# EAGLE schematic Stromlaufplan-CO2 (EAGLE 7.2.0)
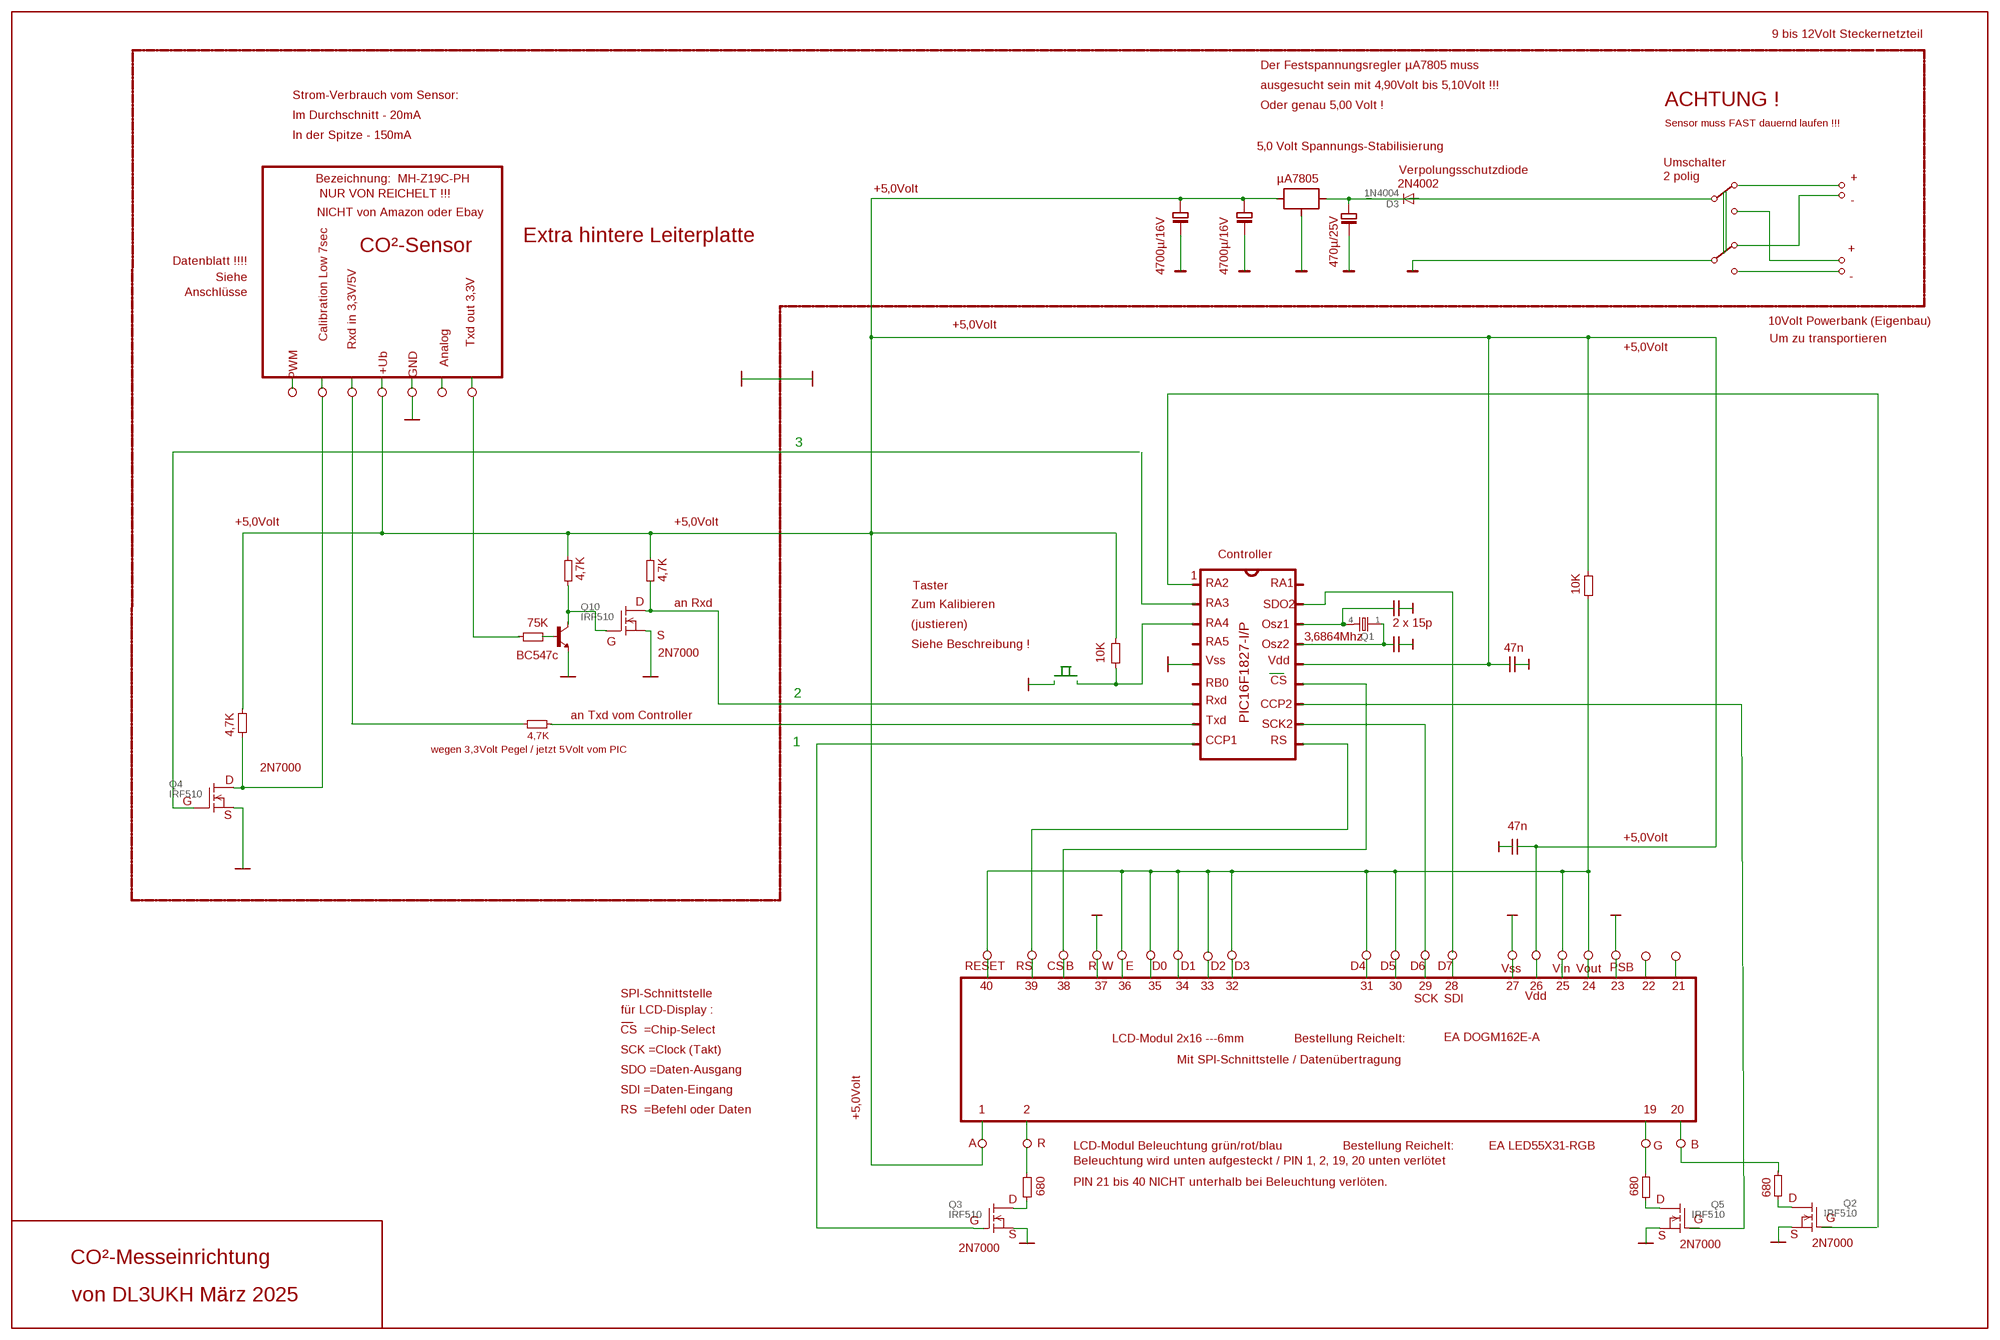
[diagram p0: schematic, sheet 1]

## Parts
D3  1N4004  [DO41-10]
Q1  86SMX  [86SMX]
Q2  IRF510  [TO220]
Q3  IRF510  [TO220]
Q4  IRF510  [TO220]
Q5  IRF510  [TO220]
Q10  IRF510  [TO220]

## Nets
N$7: Q4.1(G)
N$21: Q10.3(S)
N$33: Q10.1(G)
N$39: Q10.2(D)
N$44: Q1.4
N$45: Q1.1
N$47: D3.C
N$56: Q3.2(D)
N$58: Q3.3(S)
N$59: Q3.1(G)
N$60: Q5.1(G)
N$61: Q5.2(D)
N$63: Q5.3(S)
N$64: Q2.2(D)
N$85: Q4.3(S)
N$86: Q4.2(D)
N$87: D3.A
N$96: Q2.3(S)
N$97: Q2.1(G)

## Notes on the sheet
- 9 bis 12Volt Steckernetzteil
- Der Festspannungsregler µA7805 muss
- ausgesucht sein mit 4,90Volt bis 5,10Volt !!!
- Strom-Verbrauch vom Sensor:
- Oder genau 5,00 Volt ! | ACHTUNG !
- Im Durchschnitt - 20mA
- Sensor muss FAST dauernd laufen !!!
- In der Spitze - 150mA
- 5,0 Volt Spannungs-Stabilisierung
- Umschalter
- Bezeichnung:  MH-Z19C-PH | Verpolungsschutzdiode
- µA7805 | 2 polig | +
- NUR VON REICHELT !!! | 2N4002
- +5,0Volt
- -
- NICHT von Amazon oder Ebay
- Calibration Low 7sec
- CO²-Sensor | Extra hintere Leiterplatte
- +
- Datenblatt !!!!
- Rxd in 3,3V/5V | 470µ/25V
- Siehe | 4700µ/16V | 4700µ/16V
- Txd out 3,3V | -
- Anschlüsse
- 10Volt Powerbank (Eigenbau)
- Analog | +5,0Volt
- Um zu transportieren
- PWM | +Ub | GND | +5,0Volt
- 3
- +5,0Volt | +5,0Volt
- Controller
- 4,7K | 4,7K | 1
- Taster | RA2 | RA1
- 10K
- D | an Rxd | Zum Kalibieren | RA3 | SDO2
- 75K | (justieren) | RA4 | Osz1 | 2 x 15p
- S | 3,6864Mhz
- G | Siehe Beschreibung ! | RA5 | Osz2
- 47n
- BC547c | 2N7000
- 10K | Vss | Vdd
- RB0 | CS
- 2
- Rxd
- CCP2
- an Txd vom Controller
- Txd | PIC16F1827-I/P
- SCK2
- 4,7K | 4,7K
- 1 | CCP1 | RS
- wegen 3,3Volt Pegel / jetzt 5Volt vom PIC
- 2N7000
- D
- G
- S | 47n
- +5,0Volt
- RESET | RS | CS | B | R | W | E | D0 | D1 | D2 | D3 | D4 | D5 | D6 | D7 | Vss | Vin | Vout | PSB
- 40 | 39 | 38 | 37 | 36 | 35 | 34 | 33 | 32 | 31 | 30 | 29 | 28 | 27 | 26 | 25 | 24 | 23 | 22 | 21
- SPI-Schnittstelle | Vdd
- SCK | SDI
- für LCD-Display :
- CS  =Chip-Select
- LCD-Modul 2x16 ---6mm | Bestellung Reichelt: | EA DOGM162E-A
- SCK =Clock (Takt)
- Mit SPI-Schnittstelle / Datenübertragung
- SDO =Daten-Ausgang
- SDI =Daten-Eingang
- RS  =Befehl oder Daten | 1 | 2 | 19 | 20
- +5,0Volt
- A | R | LCD-Modul Beleuchtung grün/rot/blau | Bestellung Reichelt: | EA LED55X31-RGB | G | B
- Beleuchtung wird unten aufgesteckt / PIN 1, 2, 19, 20 unten verlötet
- PIN 21 bis 40 NICHT unterhalb bei Beleuchtung verlöten.
- 680 | 680 | 680
- D | D | D
- G | G | G
- S | S | S
- 2N7000 | 2N7000
- 2N7000
- CO²-Messeinrichtung
- von DL3UKH März 2025

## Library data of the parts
D3 = diode:1N4004: DIODE
Q1 = crystal:86SMX: CRYSTAL
Q2-Q5 Q10 = transistor-fet:IRF510: N-Channel Enhancement MOSFET (HEXFET); 100V; 5,6A; 0,54Ohm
